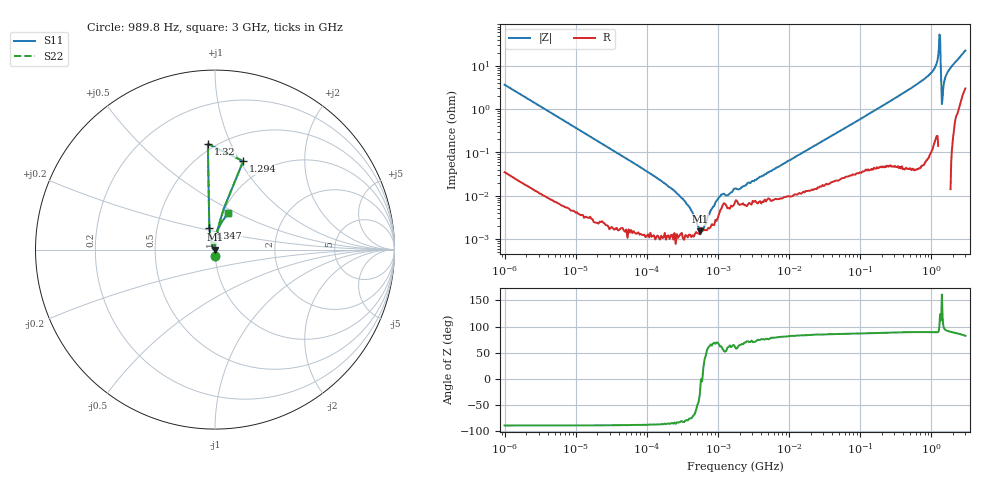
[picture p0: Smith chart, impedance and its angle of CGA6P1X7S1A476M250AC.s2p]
! S-Parameter Data Generated by TDK Corporation
! Copyright(C) 2019 TDK Corporation.
! All Rights Reserved.
! TDK P/N: CGA6P1X7S1A476M250AC (Multilayer Ceramic Chip Capacitor)
! Property: C=47uF
! Size(LxWxT): 3.2x2.5x2.5mm
! Model Type: s2p (Touchstone File Format Version 1.0)
! Frequency: DC=Yes Start=0.000989846MHz Stop=3000MHz 463points Log-sweep
! Model Generated on July 26, 2019
! Port Assignments:
!  1 ---| |--- 2
! Applicable Conditions:
!  Temperature = 25 degC
!  DC Bias Voltage = 0 V
!  Small Signal Operation
! Terms and conditions regarding TDK Simulation Models
! (1)This simulation model is being provided solely for informational purposes. Please refer to the specifications of the products in terms of detailed characteristics of such products.
! (2)In no event shall TDK Corporation of any of its subsidiaries be liable for any loss or damage arising, directly or indirectly,
!  From any information contained in this simulation model, including, but not limited to loss or damages arising from any inaccuracies, omissions or errors in connection with such information.
! (3)Any and all copyrights on this simulation model are owned by TDK Corporation.
!  Duplication or redistribution of this simulation model without prior written permission from TDK Corporation is prohibited.
! (4)This simulation model is subject to any modification or change without any prior notice.
! (5)Neither TDK Corporation nor any of its subsidiaries shall make any warranty, express or implied,
!  Including but not limited to the correctness, implied warranties of merchantability and fitness for a particular purpose with respect to this simulation models.
! (6)The use of this simulation model shall be deemed to have consented to the terms and conditions hereof.
# Hz S MA R 50
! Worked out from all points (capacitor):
!   462 points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, 989.8 Hz to 3 GHz, reference 50 ohm
!   read as one part in series: C = 43.9 uF near 1.07 kHz
!   lowest |Z| = 1.49 mohm at 550.5 kHz (marker M1)
!   series resonance near 599.8 kHz, so ESL is about 1.6 nH
!   S11 on the Smith chart (normalised r, x): 989.8 Hz: 1.00, -0.07; 1.294 GHz: 0.77, +1.03; 1.32 GHz: 0.46, +0.82; 1.347 GHz: 0.91, +0.22; 3 GHz: 1.06, +0.45
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989.846  0.0365 -87.4  0.999 2.1  0.999 2.1  0.0365 -87.4
12024.64  0.003059 -89.1  1 0.2  1 0.2  0.003059 -89.1
146075.1  0.0002401 -87.4  1 0.0  1 0.0  0.0002401 -87.4
283561.7  0.0001013 -83.3  1 0.0  1 0.0  0.0001013 -83.3
550451.5  1.494e-05 -31.3  1 0.0  1 0.0  1.494e-05 -31.3
1350401  0.0001012 59.4  0.9999 -0.0  0.9999 -0.0  0.0001012 59.4
1774518  0.0001479 57.6  0.9999 -0.0  0.9999 -0.0  0.0001479 57.6
2.073191e7  0.001307 83.8  0.9999 -0.1  0.9999 -0.1  0.001307 83.8
2.507343e8  0.01458 87.3  0.9994 -0.8  0.9994 -0.8  0.01458 87.3
9.779672e8  0.06707 85.3  0.9968 -3.8  0.9968 -3.8  0.06707 85.3
1.171007e9  0.1074 82.6  0.9919 -6.2  0.9919 -6.2  0.1074 82.6
1.218836e9  0.1367 81.2  0.9882 -7.9  0.9882 -7.9  0.1367 81.2
1.268618e9  0.2333 77.9  0.9781 -13.5  0.9781 -13.5  0.2333 77.9
1.294266e9  0.5171 72.3  0.9765 -30.3  0.9765 -30.3  0.5171 72.3
1.320433e9  0.5906 93.9  1.195 -29.5  1.195 -29.5  0.5906 93.9
1.347129e9  0.1232 104.8  1.038 -6.6  1.038 -6.6  0.1232 104.8
1.402151e9  0.01323 160.9  1.013 -0.2  1.013 -0.2  0.01323 160.9
1.430499e9  0.01743 119.9  1.009 -0.9  1.009 -0.9  0.01743 119.9
1.45942e9  0.02869 102.2  1.006 -1.6  1.006 -1.6  0.02869 102.2
1.54974e9  0.05135 91.3  1.002 -2.9  1.002 -2.9  0.05135 91.3
1.67892e9  0.07026 87.5  0.9994 -4.0  0.9994 -4.0  0.07026 87.5
3e9  0.2147 70.1  0.9486 -12.3  0.9486 -12.3  0.2147 70.1
